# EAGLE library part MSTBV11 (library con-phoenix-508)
PHOENIX
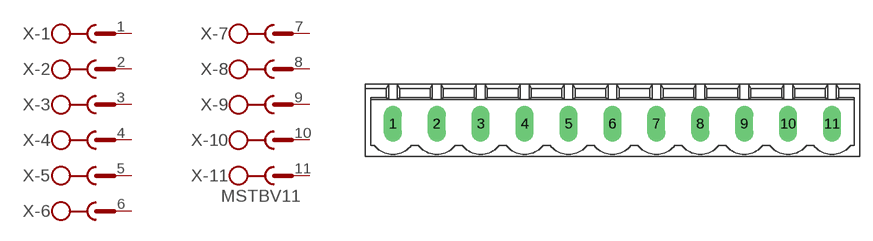
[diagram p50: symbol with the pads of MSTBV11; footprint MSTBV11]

Designator prefix X; gates -1=SK -2=SK -3=SK -4=SK -5=SK -6=SK -7=SK -8=SK -9=SK -10=SK -11=SKV

## MSTBV11 (OC_FARNELL: unknown; OC_NEWARK: unknown)  [MSTBV11]
1  -1:1  pas
2  -2:1  pas
3  -3:1  pas
4  -4:1  pas
5  -5:1  pas
6  -6:1  pas
7  -7:1  pas
8  -8:1  pas
9  -9:1  pas
10  -10:1  pas
11  -11:1  pas

## Footprint MSTBV11 (pad centres in mm)
PHOENIX
drill 1.397 long: 1 -25.4,0; 2 -20.32,0; 3 -15.24,0; 4 -10.16,0; 5 -5.08,0; 6 0,0; 7 5.08,0; 8 10.16,0; 9 15.24,0; 10 20.32,0; 11 25.4,0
